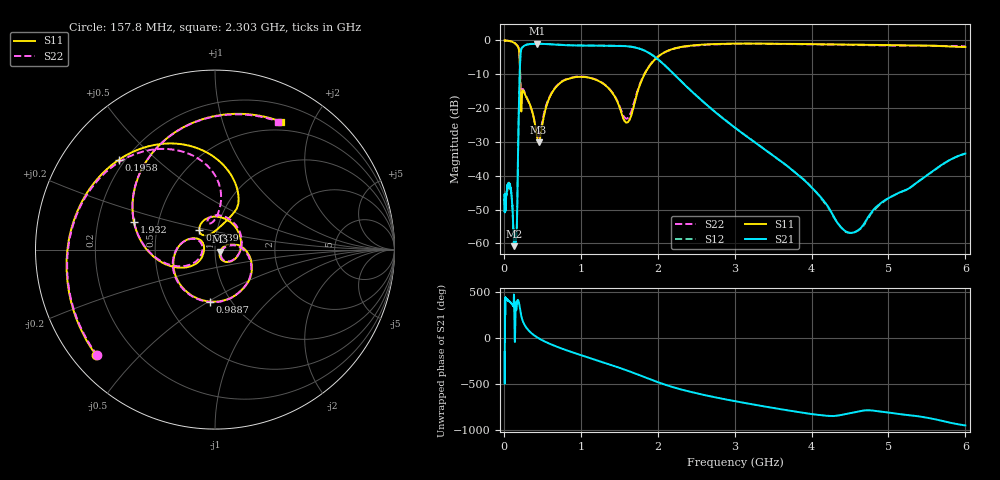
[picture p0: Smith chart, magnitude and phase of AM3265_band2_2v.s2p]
!Agilent Technologies,E8364B,MY43040894,A.07.50.67
!Agilent E8364B: A.07.50.67
!Date: Friday, May 09, 2025 07:23:05
!Correction: S11(Full 2 Port(1,2))
!S21(Full 2 Port(1,2))
!S12(Full 2 Port(1,2))
!S22(Full 2 Port(1,2))
!S2P File: Measurements: S11, S21, S12, S22:Log Frequency Sweep
# Hz S  dB  R 50
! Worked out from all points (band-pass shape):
!   3201 points, 10 MHz to 6 GHz, reference 50 ohm
!   highest |S21| = -0.98 dB at 431.3 MHz (marker M1); lowest = -60.8 dB at 137.7 MHz (marker M2)
!   |S21| within 3 dB of the highest: 217.5 MHz to 1.907 GHz (1.69 GHz wide, 159 % of centre)
!   lowest |S11| = -30.1 dB at 451.6 MHz (marker M3), VSWR 1.06, Z = 53 - j1.17 ohm
!   |S11| at or under -10 dB: 210.7 MHz to 1.828 GHz (1.617 GHz wide, 159 % of centre)
!   |S22| runs from -28.4 to 0.0 dB; largest |S21 - S12| = 0.01
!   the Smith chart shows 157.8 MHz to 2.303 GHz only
!   S11 on the Smith chart (normalised r, x): 157.8 MHz: 0.07, -0.38; 195.8 MHz: 0.18, +0.38; 233.9 MHz: 0.82, +0.18; 988.7 MHz: 0.80, -0.51; 1.932 GHz: 0.36, +0.15; 2.303 GHz: 0.39, +1.57
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1e7  0.01 -7.1  -45.99 -151.8  -45.95 -119.7  -0.07 -6.8
2.908064e7  -0.03 -19.7  -46.86 72.1  -46.50 74.3  -0.04 -19.7
8.439949e7  -0.18 -60.4  -43.24 32.7  -43.52 30.7  -0.22 -60.7
1.377343e8  -0.69 -112.1  -60.79 151.7  -57.94 -168.4  -0.73 -111.9
1.577894e8  -1.05 -138.7  -58.10 -6.4  -58.01 -77.9  -1.09 -138.0
1.958125e8  -2.70 136.8  -19.65 27.2  -19.62 27.1  -2.63 142.3
2.339417e8  -17.10 128.7  -2.21 -142.7  -2.17 -142.7  -15.56 104.6
2.44949e8  -14.76 97.1  -1.94 -170.5  -1.90 -170.6  -14.33 84.9
3.113553e8  -17.57 -13.7  -1.17 94.6  -1.13 94.6  -17.56 -13.2
4.31289e8  -28.58 -45.7  -0.98 10.9  -0.94 10.8  -27.53 -38.4
4.515817e8  -30.09 -20.6  -0.98 0.5  -0.95 0.5  -28.42 -17.7
7.123273e8  -12.96 -24.0  -1.27 -99.4  -1.23 -99.4  -12.83 -27.6
9.886894e8  -10.72 -95.5  -1.49 -179.8  -1.46 -179.8  -10.64 -97.9
1.353203e9  -13.92 174.3  -1.54 81.1  -1.51 81.1  -13.86 174.4
1.931513e9  -6.41 160.9  -4.34 -95.4  -4.31 -95.4  -6.35 160.3
2.067357e9  -3.78 121.4  -6.83 -136.3  -6.80 -136.3  -3.79 121.7
2.303015e9  -1.91 62.8  -12.04 164.0  -12.02 164.0  -1.98 63.7
3.202913e9  -0.90 -91.5  -29.12 6.1  -29.08 6.0  -0.98 -91.5
3.818953e9  -1.02 -178.3  -39.60 -80.6  -39.55 -81.2  -1.08 -179.7
4.490206e9  -1.22 91.9  -56.79 -95.8  -56.86 -96.5  -1.30 90.5
5.185309e9  -1.41 1.1  -44.56 -108.3  -44.55 -107.6  -1.53 1.2
6e9  -1.93 -97.0  -33.43 132.4  -33.41 132.5  -1.69 -96.5
